| ussxh8g80bc.ibs * IBIS 4.2 Model
| 8Gb DDR3L SDRAM
| This Model is valid for Commercial Temperature Range 0C<=Tc<=85C
| Valid for DDR3L-1066/1333/1600/1866 operation
[IBIS Ver]   4.2
[File Name]   ussxh8g80bc.ibs
[Date]   02/12/2019
[File Rev]   2.0
| COMPONENT: SCB13(15)H8G802BF (78-Ball FBGA, x8, 7.5mm X 10.6mm)
[Component]   SCB13(15)H8G802BF
[Manufacturer]  UniIC Semiconductors Corp.
[Package]
|   typ   min   max
R_pkg   274.7m   193.6m   372.7m
L_pkg   1.708nH   1.077nH   2.475nH
C_pkg   0.413pF   0.333pF   0.645pF
[Pin]   signal_name  model_name   R_pin   L_pin   C_pin
A1   VSS   GND
A2   VDD   POWER
A3   NC   NC
A7   NF_TDQS#   NF_TDQS#
A8   VSS   GND
A9   VDD   POWER
B1   VSS   GND
B2   VSSQ   GND
B3   DQ0   DQ
B7   DM_TDQS   DM_TDQS
B8   VSSQ   GND
B9   VDDQ   POWER
C1   VDDQ   POWER
C2   DQ2   DQ
C3   DQS   DQS
C7   DQ1   DQ
C8   DQ3   DQ
C9   VSSQ   GND
D1   VSSQ   GND
D2   DQ6   DQ
D3   DQS#   DQS
D7   VDD   POWER
D8   VSS   GND
D9   VSSQ   GND
E1   VREFDQ   POWER
E2   VDDQ   POWER
E3   DQ4   DQ
E7   DQ7   DQ
E8   DQ5   DQ
E9   VDDQ   POWER
F1   NC   NC
F2   VSS   GND
F3   RAS#   INPUT
F7   CK   CLKIN
F8   VSS   GND
F9   NC   NC
G1   ODT   INPUT
G2   VDD   POWER
G3   CAS#   INPUT
G7   CK#   CLKIN
G8   VDD   POWER
G9   CKE   INPUT
H1   NC   NC
H2   CS#   INPUT
H3   WE#   INPUT
H7   A10   INPUT
H8   ZQ   NC
H9   NC   NC
J1   VSS   GND
J2   BA0   INPUT
J3   BA2   INPUT
J7   A15   INPUT
J8   VREFCA   POWER
J9   VSS   GND
K1   VDD   POWER
K2   A3   INPUT
K3   A0   INPUT
K7   A12   INPUT
K8   BA1   INPUT
K9   VDD   POWER
L1   VSS   GND
L2   A5   INPUT
L3   A2   INPUT
L7   A1   INPUT
L8   A4   INPUT
L9   VSS   GND
M1   VDD   POWER
M2   A7   INPUT
M3   A9   INPUT
M7   A11   INPUT
M8   A6   INPUT
M9   VDD   POWER
N1   VSS   GND
N2   RESET#   RESET
N3   A13   INPUT
N7   A14   INPUT
N8   A8   INPUT
N9   VSS   GND
|***********************PIN MAPPING*****************************************
[Pin Mapping] pulldown_ref pullup_ref gnd_clamp_ref power_clamp_ref ext_ref
A1   VSS   NC
A2   NC   VDD
A3   NC   NC
A7   VSS   VDDQ   VSS   VDDQ
A8   VSS   NC
A9   NC   VDD
B1   VSS   NC
B2   VSS   NC
B3   VSS   VDDQ   VSS   VDDQ
B7   VSS   VDDQ   VSS   VDDQ
B8   VSS   NC
B9   NC   VDDQ
C1   NC   VDDQ
C2   VSS   VDDQ   VSS   VDDQ
C3   VSS   VDDQ   VSS   VDDQ
C7   VSS   VDDQ   VSS   VDDQ
C8   VSS   VDDQ   VSS   VDDQ
C9   VSS   NC
D1   VSS   NC
D2   VSS   VDDQ   VSS   VDDQ
D3   VSS   VDDQ   VSS   VDDQ
D7   NC   VDD
D8   VSS   NC
D9   VSS   NC
E1   NC   VREFDQ
E2   NC   VDDQ
E3   VSS   VDDQ   VSS   VDDQ
E7   VSS   VDDQ   VSS   VDDQ
E8   VSS   VDDQ   VSS   VDDQ
E9   NC   VDDQ
F1   NC   NC
F2   VSSL   NC
F3   NC   NC   VSS   VDD
F7   NC   NC   VSS   VDD
F8   VSS   NC
F9   NC   NC
G1   NC   NC   VSS   VDD
G2   NC   VDDL
G3   NC   NC   VSS   VDD
G7   NC   NC   VSS   VDD
G8   NC   VDD
G9   NC   NC   VSS   VDD
H1   NC   NC
H2   NC   NC   VSS   VDD
H3   NC   NC   VSS   VDD
H7   NC   NC   VSS   VDD
H8   NC   NC
H9   NC   NC
J1   VSS   NC
J2   NC   NC   VSS   VDD
J3   NC   NC   VSS   VDD
J7   NC   NC   VSS   VDD
J8   NC   VREFCA
J9   VSS   NC
K1   NC   VDD
K2   NC   NC   VSS   VDD
K3   NC   NC   VSS   VDD
K7   NC   NC   VSS   VDD
K8   NC   NC   VSS   VDD
K9   NC   VDD
L1   VSS   NC
L2   NC   NC   VSS   VDD
L3   NC   NC   VSS   VDD
L7   NC   NC   VSS   VDD
L8   NC   NC   VSS   VDD
L9   VSS   NC
M1   NC   VDD
M2   NC   NC   VSS   VDD
M3   NC   NC   VSS   VDD
M7   NC   NC   VSS   VDD
M8   NC   NC   VSS   VDD
M9   NC   VDD
N1   VSS   NC
N2   NC   NC   VSS   VDD
N3   NC   NC   VSS   VDD
N7   NC   NC   VSS   VDD
N8   NC   NC   VSS   VDD
N9   VSS   NC
|**********************DIFF PIN*********************************************
[Diff_pin]   inv_pin   vdiff   tdelay_typ   tdelay_min   tdelay_max
   C3   D3   0.320V   0ns   NA   NA
   F7   G7   0.320V   0ns   NA   NA
|   Model Selector
[Model Selector] DQ
DQ_34   34 Ohm Data I/O with no ODT, 800-2133Mbps
DQ_40   40 Ohm Data I/O with no ODT, 800-2133Mbps
DQ_IN_ODT20   Data Input with 20ohm ODT, 800-2133Mbps
DQ_IN_ODT30   Data Input with 30ohm ODT, 800-2133Mbps
DQ_IN_ODT40   Data Input with 40ohm ODT, 800-2133Mbps
DQ_IN_ODT60   Data Input with 60ohm ODT, 800-2133Mbps
DQ_IN_ODT120  Data Input with 120ohm ODT, 800-2133Mbps
[Model Selector] DQS
DQS_34   34 Ohm Data Strobe I/O with no ODT, 800-2133Mbps
DQS_40   40 Ohm Data Strobe I/O with no ODT, 800-2133Mbps
DQS_IN_ODT20  Data Strobe Input with 20ohm ODT, 800-2133Mbps
DQS_IN_ODT30  Data Strobe Input with 30ohm ODT, 800-2133Mbps
DQS_IN_ODT40  Data Strobe Input with 40ohm ODT, 800-2133Mbps
DQS_IN_ODT60  Data Strobe Input with 60ohm ODT, 800-2133Mbps
DQS_IN_ODT120 Data Strobe Input with 120ohm ODT, 800-2133Mbps
[Model Selector] DM
DM_INPUT   DM Input Model with no ODT, 800-2133Mbps
DM_ODT20   DM Input Model with 20ohm ODT, 800-2133Mbps
DM_ODT30   DM Input Model with 30ohm ODT, 800-2133Mbps
DM_ODT40   DM Input Model with 40ohm ODT, 800-2133Mbps
DM_ODT60   DM Input Model with 60ohm ODT, 800-2133Mbps
DM_ODT120   DM Input Model with 120ohm ODT, 800-2133Mbps
[Model Selector] DM_TDQS
DM_INPUT   DM Input Model with no ODT, 800-2133Mbps
DM_ODT20   DM Input Model with 20ohm ODT, 800-2133Mbps
DM_ODT30   DM Input Model with 30ohm ODT, 800-2133Mbps
DM_ODT40   DM Input Model with 40ohm ODT, 800-2133Mbps
DM_ODT60   DM Input Model with 60ohm ODT, 800-2133Mbps
DM_ODT120   DM Input Model with 120ohm ODT, 800-2133Mbps
TDQS_ODT20   TDQS Terminator Model with 20ohm ODT, 800-2133Mbps
TDQS_ODT30   TDQS Terminator Model with 30ohm ODT, 800-2133Mbps
TDQS_ODT40   TDQS Terminator Model with 40ohm ODT, 800-2133Mbps
TDQS_ODT60   TDQS Terminator Model with 60ohm ODT, 800-2133Mbps
TDQS_ODT120   TDQS Terminator Model with 120ohm ODT, 800-2133Mbps
[Model Selector] NF_TDQS#
NF_INPUT   Non-Functioning Terminator Model
TDQS_ODT20   TDQS Terminator Model with 20ohm ODT, 800-2133Mbps
TDQS_ODT30   TDQS Terminator Model with 30ohm ODT, 800-2133Mbps
TDQS_ODT40   TDQS Terminator Model with 40ohm ODT, 800-2133Mbps
TDQS_ODT60   TDQS Terminator Model with 60ohm ODT, 800-2133Mbps
TDQS_ODT120   TDQS Terminator Model with 120ohm ODT, 800-2133Mbps
| Sparse Matrix Package Model for SCB13(15)H8G802BF_78ball_pkg (x8)
[Define Package Model]  KTC_8G3D_x8_RDL_DDP_PKG
[Manufacturer]  UniIC Semiconductors Corp.
[OEM]  UniIC
[Description]  None
[Number Of Pins]  41
[Pin Numbers]
|Pin Num   Terminal Name
K3   | A0:A0_D2Pad_78
L7   | A1:A1_D2Pad_83
L3   | A2:A2_D2Pad_82
K2   | A3:A3_D2Pad_74
L8   | A4:A4_D2Pad_79
L2   | A5:A5_D2Pad_80
M8   | A6:A6_D2Pad_81
M2   | A7:A7_D2Pad_84
N8   | A8:A8_D2Pad_85
M3   | A9:A9_D2Pad_86
H7   | A10:A10_D2Pad_65
M7   | A11:A11_D2Pad_87
K7   | A12:A12_D2Pad_75
N3   | A13:A13_D2Pad_88
N7   | A14:A14_D2Pad_89
J7   | A15:A15_D2Pad_73
J2   | BA0:BA0_D2Pad_70
K8   | BA1:BA1_D2Pad_71
J3   | BA2:BA2_D2Pad_72
G3   | CASB:CASB_D2Pad_62
F7   | CK:CK_D2Pad_57
G7   | CKB:CKB_D2Pad_58
G9   | CKE:CKE_D2Pad_59
H2   | CSB:CSB_D2Pad_63
B7   | DML:DML_D2Pad_30
A7   | DMU:DMU_D2Pad_26
B3   | DQL0:DQL0_D1Pad_32
C7   | DQL1:DQL1_D1Pad_34
C2   | DQL2:DQL2_D1Pad_36
C8   | DQL3:DQL3_D1Pad_38
E3   | DQL4:DQL4_D2Pad_32
E8   | DQL5:DQL5_D2Pad_34
D2   | DQL6:DQL6_D2Pad_36
E7   | DQL7:DQL7_D2Pad_38
C3   | DQSL:DQSL_D2Pad_40
D3   | DQSLB:DQSLB_D2Pad_41
G1   | ODT:ODT_D2Pad_61
F3   | RASB:RASB_D2Pad_60
N2   | RESETB:RESETB_D2Pad_92
H3   | WEB:WEB_D2Pad_64
H8   | ZQ:ZQ_D2Pad_69
[Model Data]
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[End Model Data]
[End Package Model]
| Models and submodels in the file (29): DQ_34 (I/O), DQ_40 (I/O), DQ_IN_ODT20 (Input), DQ_IN_ODT30 (Input), DQ_IN_ODT40 (Input), DQ_IN_ODT60 (Input), DQ_IN_ODT120 (Input), DQS_34 (I/O), DQS_40 (I/O), DQS_IN_ODT20 (Input), DQS_IN_ODT30 (Input), DQS_IN_ODT40 (Input), DQS_IN_ODT60 (Input), DQS_IN_ODT120 (Input), DM_INPUT (Input), DM_ODT20 (Input), DM_ODT30 (Input), DM_ODT40 (Input), DM_ODT60 (Input), DM_ODT120 (Input), TDQS_ODT20 (Terminator), TDQS_ODT30 (Terminator), TDQS_ODT40 (Terminator), TDQS_ODT60 (Terminator), TDQS_ODT120 (Terminator), INPUT (Input), CLKIN (Input), RESET (Input), NF_INPUT (Terminator)
